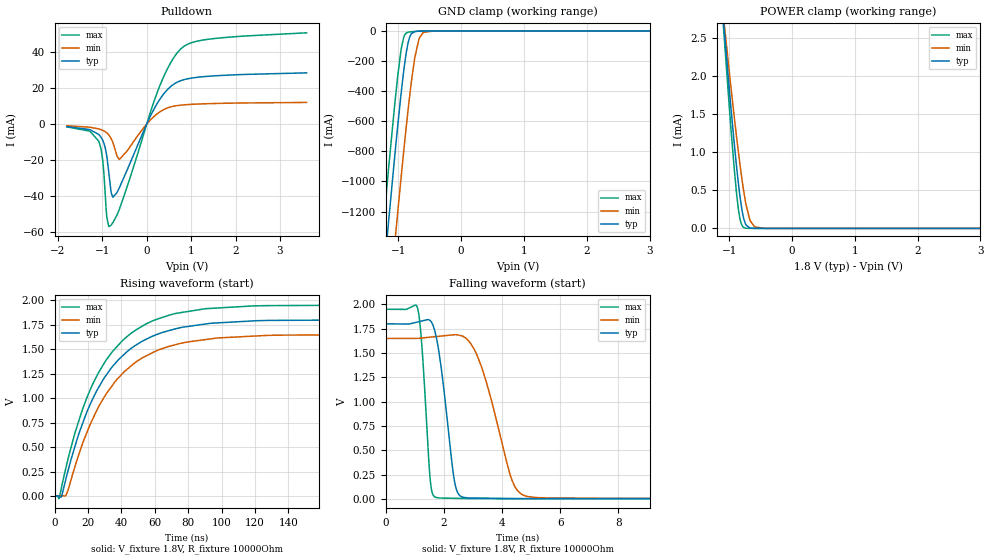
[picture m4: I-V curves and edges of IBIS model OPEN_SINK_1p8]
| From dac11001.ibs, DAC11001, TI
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|   OPEN_SINK_1p8 Model
[Model]   OPEN_SINK_1p8
Model_type   Open_sink
Polarity   Non-Inverting
Vmeas = 0.9
Vref = 1.8
Cref = 2pF
Rref = 10000
|   typ   min   max
C_comp   0.981pF   0.976pF   0.99pF
[Voltage Range]   1.8   1.65   1.95
[Temperature Range]   25   125   -40
[Pullup Reference]   1.8   1.65   1.95
[Pulldown Reference]   0   -0   0
[Power Clamp Reference]   1.8   1.65   1.95
[GND Clamp Reference]   0   0   0
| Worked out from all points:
|   slope of the pulldown table from 0 to 0.27 V, typ, clamps not added: 21.1 ohm
|   GND clamp passes 1 mA (typ) near -0.68 V on its own axis
|   POWER clamp passes 1 mA (typ) near -0.91 V on its own axis
|   falling waveform, V_fixture 1.8V, R_fixture 10000Ohm: 20-80 % time 418ps typ, 865ps min, 236ps max; typ from 1.8 V to 0.003 V
|   rising waveform, V_fixture 1.8V, R_fixture 10000Ohm: 20-80 % time 31.7ns typ, 32.6ns min, 31.1ns max; typ from 0.003 V to 1.8 V
[Pulldown]
|   Voltage   I(typ)   I(min)   I(max)
-1.8V     -1.392mA   -925uA     -1.562mA
-1.082V   -5.757mA   -2.672mA   -9.449mA
-995.4mV  -8.774mA   -3.416mA   -19.21mA
-898.2mV  -17.89mA   -4.888mA   -51.94mA
-849.6mV  -27.86mA   -6.13mA    -56.99mA
-763.2mV  -40.55mA   -10.16mA   -54.83mA
-671.4mV  -38.14mA   -17.54mA   -50.63mA
-617.4mV  -35.46mA   -19.68mA   -47.47mA
230.4mV   11.26mA    5.588mA    17.17mA
765mV     24.13mA    10.52mA    41.76mA
1.37V     26.55mA    11.34mA    47.1mA
3.6V      28.48mA    12.04mA    50.74mA
[GND Clamp]
|   Voltage   I(typ)   I(min)   I(max)
-1.8V     -4.34A     -4.922A    -3.994A
-1.433V   -2.571A    -3.162A    -2.218A
-1.206V   -1.506A    -2.099A    -1.15A
-1.179V   -1.382A    -1.974A    -1.027A
-1.157V   -1.284A    -1.875A    -929mA
-1.055V   -827.3mA   -1.411A    -482.9mA
-1.012V   -643.7mA   -1.22A     -312mA
-952.2mV  -406.3mA   -963.2mA   -118.2mA
-871.2mV  -140.2mA   -630.9mA   -13.18mA
-736.2mV  -3.489mA   -175.7mA   -2.778mA
-601.2mV  -180.3uA   -9.228mA   -333.6uA
3.6V      0A         0A         0A
[POWER Clamp]
|   Voltage   I(typ)   I(min)   I(max)
-1.8V     9.999mA    8.694mA    11.2mA
-1.157V   3.371mA    3.315mA    3.403mA
-990mV    1.753mA    1.995mA    1.506mA
-914.4mV  1.078mA    1.432mA    741uA
-860.4mV  644.8uA    1.053mA    301.5uA
-817.2mV  354.7uA    771.2uA    88.9uA
-768.6mV  129.8uA    489.2uA    12.07uA
-730.8mV  43.96uA    307.5uA    2.051uA
-666mV    4.546uA    102uA      85.51nA
-595.8mV  324.2nA    19.73uA    0A
-444.6mV  0A         296.1nA    0A
3.6V      0A         0A         0A
[Ramp]
R_load = 10000
|   typ   min   max
dV/dt_r   1.07809/3.15691e-08   0.986607/3.24264e-08   1.16859/3.09578e-08
dV/dt_f   1.07809/4.1613e-10   0.986607/8.63662e-10   1.16859/2.36058e-10
[Falling Waveform]
V_fixture = 1.8V
V_fixture_min = 1.65V
V_fixture_max = 1.95V
R_fixture = 10000Ohm
C_fixture = 0F
|   Time   V(typ)   V(min)   V(max)
0s        1.8V       1.65V      1.95V
1.106ns   1.82V      1.651V     1.952V
1.525ns   1.834V     1.663V     221.4mV
1.617ns   1.795V     1.666V     49.84mV
1.892ns   1.387V     1.674V     9.378mV
2.403ns   130.6mV    1.689V     6.284mV
3.013ns   9.391mV    1.556V     2.591mV
4.539ns   3.503mV    84.55mV    2.591mV
7.793ns   3.503mV    6.159mV    2.591mV
3.5us     3.191mV    5.649mV    2.356mV
[Rising Waveform]
V_fixture = 1.8V
V_fixture_min = 1.65V
V_fixture_max = 1.95V
R_fixture = 10000Ohm
C_fixture = 0F
|   Time   V(typ)   V(min)   V(max)
0s        3.191mV    5.649mV    2.356mV
2.596ns   -1.234mV   4.301mV    -21.88mV
4.059ns   -2.3mV     3.542mV    90.76mV
6.731ns   178.8mV    9.413mV    292.1mV
12.38ns   522.9mV    316.9mV    659.9mV
21.21ns   936.1mV    732mV      1.084V
40.28ns   1.425V     1.244V     1.581V
68.43ns   1.688V     1.527V     1.845V
118.7ns   1.787V     1.632V     1.94V
3.5us     1.8V       1.65V      1.95V
